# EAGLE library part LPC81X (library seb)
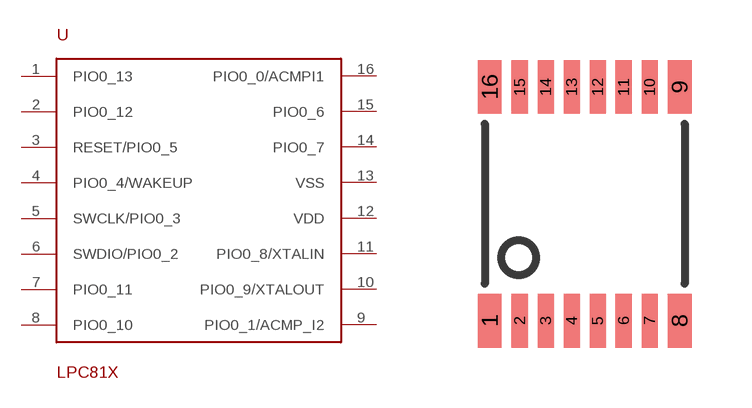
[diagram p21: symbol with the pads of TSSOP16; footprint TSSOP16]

Designator prefix -

## LPC81X  [TSSOP16]
1  PIO0_13
2  PIO0_12
3  RESET/PIO0_5
4  PIO0_4/WAKEUP
5  SWCLK/PIO0_3
6  SWDIO/PIO0_2
7  PIO0_11
8  PIO0_10
9  PIO0_1/ACMP_I2
10  PIO0_9/XTALOUT
11  PIO0_8/XTALIN
12  VDD
13  VSS
14  PIO0_7
15  PIO0_6
16  PIO0_0/ACMPI1

## Footprint TSSOP16 (pad centres in mm)
smd 0.6 x 1.35: 1 -2.375,-2.925; 8 2.375,-2.925; 9 2.375,2.925; 16 -2.375,2.925
smd 0.4 x 1.35: 2 -1.625,-2.925; 3 -0.975,-2.925; 4 -0.325,-2.925; 5 0.325,-2.925; 6 0.975,-2.925; 7 1.625,-2.925; 10 1.625,2.925; 11 0.975,2.925; 12 0.325,2.925; 13 -0.325,2.925; 14 -0.975,2.925; 15 -1.625,2.925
